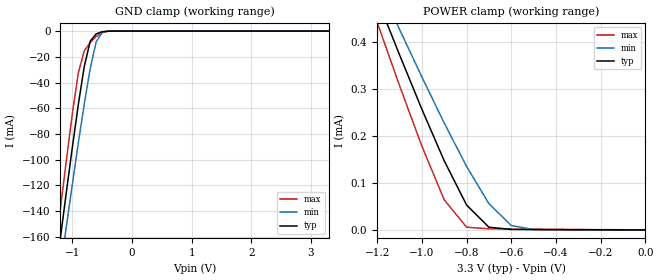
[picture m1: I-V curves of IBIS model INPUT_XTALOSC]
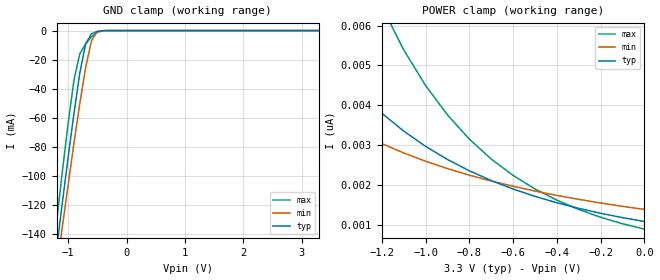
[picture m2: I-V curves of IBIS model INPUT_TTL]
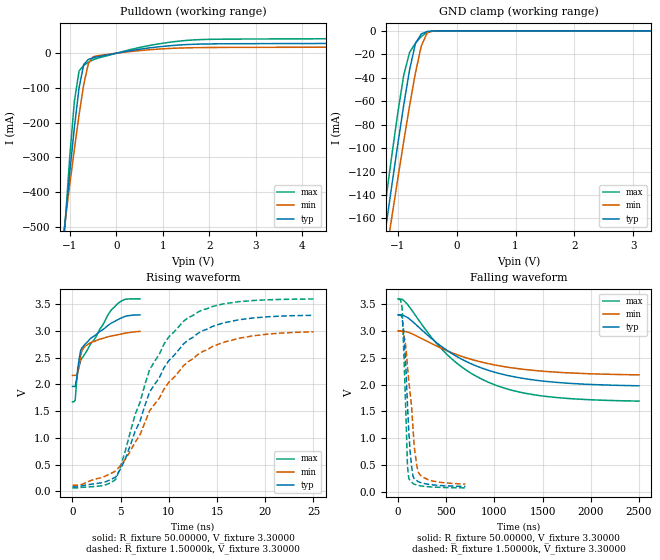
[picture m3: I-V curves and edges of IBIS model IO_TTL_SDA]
| IBIS file 5V19EE404.ibs created by s2ibis2 version 1.2
| North Carolina State University Electronics Research Laboratory  1995
[IBIS ver]   4.1
[File name]   5v19ee404.ibs
[File Rev]   2.7
[Date]   Aug 5, 2013
[Source]   IDT
[Notes]   1. Temp typ=25C, min=85C, max=-40C
[Disclaimer]
READ THESE TERMS AND CONDITIONS CAREFULLY BEFORE USING THIS IBIS MODEL.  BY
USING THIS IBIS MODEL, YOU ARE ACCEPTING AND AGREEING TO THESE TERMS AND
CONDITIONS OF USE.
Integrated Device Technology, Inc. ("IDT") hereby grants the user of this
IBIS model ("User") a non-exclusive, nontransferable license to use this
IBIS model under the following terms: The User is granted this license only
to use the IBIS model for demonstration purposes only and is not granted
rights to sell, copy (except as needed to run the IBIS model), rent, lease
or sub-license (except for demonstration) the IBIS model in whole or in
part, or in modified form to anyone. The User may modify the IBIS model to
suit its specific applications, but  rights to derivative works and such
modifications shall belong to IDT.
THIS IBIS MODEL IS PROVIDED ON AN AS IS" BASIS AND IDT  MAKES ABSOLUTELY NO
WARRANTY WITH RESPECT TO THE INFORMATION CONTAINED HEREIN.  IDT DISCLAIMS
AND USER WAIVES ALL WARRANTIES, EXPRESS AND IMPLIED, INCLUDING WARRANTIES OF
MERCHANTABILITY AND FITNESS FOR A PARTICULAR PURPOSE.  THE ENTIRE RISK AS TO
QUALITY AND PERFORMANCE IS WITH THE USER  ACCORDINGLY, IN NO EVENT SHALL IDT
BE LIABLE FOR ANY DIRECT OR INDIRECT DAMAGES, WHETHER IN CONTRACT OR TORT,
INCLUDING ANY LOST PROFITS OR OTHER INCIDENTAL, CONSEQUENTIAL, EXEMPLARY, OR
PUNITIVE DAMAGES ARISING OUT OF THE USE OR APPLICATION OF THE  IBIS MODEL,
WHETHER OR NOT IDT HAD NOTICE OF SUCH DAMAGES.
IDT reserves the right to make changes without notice to any product herein
to improve reliability, function, or design. IDT does not convey any license
under patent rights or any other intellectual property rights, including
those of third parties. IDT is not obligated to provide  maintenance or
support for the licensed IBIS model.
This model is for  IDT5V19EE404 IDT Programmable Clock
[Copyright]
Copyright 2002, Integrated Device Technology, Inc. All rights  reserved.
|History
|Rev 2.7 Updated on August 05, 2013   update RRef for TTL_SDA model
|Rev 2.6 Updated on Nov 01, 2012   update out4/4b 5/5b and single end output
|Rev 2.5 Updated on August 07, 2012   update diff table
|Rev 2.4 Updated on August 06, 2012   correct HCSL data error
|Rev 2.3 Updated on August 05, 2012   fix lvmos_1v8_s10 data error
|Rev 2.2 Updated on August 03, 2012   add lvcmos 1v8 output data
|Rev 2.1 Updated on August 02, 2012
|Rev 2.0 Updated on July 27, 2012
|Rev 1.0 Created on May 21, 2009
|   Component IDT5V19EE404
[Component]   IDT5V19EE404
[Manufacturer]   Integrated Device Technology Inc.
[Package]
| Following package parameters are for the 32 pin QFN package
| variable   typ   min   max
R_pkg   72.4655m   58.886m   86.045m
L_pkg   1.47175nH   1.11650nH   1.77850nH
C_pkg   0.07747pF   0.07444pF   0.08050pF
[Pin]  signal_name   model_name
1 vIN   POWER
2 XOUT   NC
3 XIN/REF   INPUT_XTALOSC
4 VDDx   POWER
5 CLKIN   INPUT_TTL
6 GND   GND
7 OUT1   lvcmos_se3
8 OUT2.   lvcmos_se3
9 VDDO1   POWER
10 VDD   POWER
11 SDAT   IO_TTL_SDA
12 SCLK   INPUT_TTL
13 CLKSEL   INPUT_TTL
14 AVDD   POWER
15 GND   GND
16 OUT6   lvcmos_se45
17 OUT3   lvcmos_se45
18 VDDO3   POWER
19 SEL2   INPUT_TTL
20 SEL1   INPUT_TTL
21 SEL0   INPUT_TTL
22 SD/OE   INPUT_TTL
23 GND   GND
24 VDD   POWER
[Diff Pin]  inv_pin  vdiff   tdelay_typ  tdelay_min  tdelay_max
11   10   0.000V   0.000s   0.000s   0.000s
15   14   0.000V   0.000s   0.000s   0.000s
[Model Selector] output_diff
output_lvds 3.3V LVDS output
output_lvpecl 3.3V LVPECL output
output_hcsl HCSL output
[Model Selector] lvcmos_se3
se3_1v8_s00 slew rate 00
se3_1v8_s01 slew rate 01
se3_1v8_s10 slew rate 10
se3_1v8_s11 slew rate 11
se3_3v3_s00 slew rate 00
se3_3v3_s01 slew rate 01
se3_3v3_s10 slew rate 10
se3_3v3_s11 slew rate 11
[Model Selector] lvcmos_se45
se45_1v8_s00 1.8v slew rate 00
se45_1v8_s01 1.8v slew rate 01
se45_1v8_s10 1.8v slew rate 10
se45_1v8_s11 1.8v slew rate 11
se45_3v3_s00 3.3v slew rate 00
se45_3v3_s01 3.3v slew rate 01
se45_3v3_s10 3.3v slew rate 10
se45_3v3_s11 3.3v slew rate 11
| Models and submodels in the file (22): INPUT_XTALOSC (Input), INPUT_TTL (Input), IO_TTL_SDA (I/O_open_drain), output_lvds (Output), output_lvpecl (Output_ECL), output_hcsl (Open_source), se45_1v8_s00 (Output), se45_1v8_s01 (Output), se45_1v8_s10 (Output), se45_1v8_s11 (Output), se45_3v3_s00 (Output), se45_3v3_s01 (Output), se45_3v3_s10 (Output), se45_3v3_s11 (Output), se3_1v8_s00 (Output), se3_1v8_s01 (Output), se3_1v8_s10 (Output), se3_1v8_s11 (Output), se3_3v3_s00 (Output), se3_3v3_s01 (Output), se3_3v3_s10 (Output), se3_3v3_s11 (Output)
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|   Model INPUT_XTALOSC
[Model]   INPUT_XTALOSC
Model_type   Input
Polarity   Non-Inverting
Vinl =  0.80000V
Vinh =  2.00000V
C_comp   4.00000pF   4.00000pF   4.00000pF
[Temperature Range]   25.00000   100.00000   -40.00000
[Voltage Range]   3.30000V   3.00000V   3.60000V
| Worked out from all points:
|   GND clamp passes 1 mA (typ) near -0.53 V on its own axis
|   POWER clamp passes 1 mA (typ) near -1.62 V on its own axis
[GND_clamp]
| voltage   I(typ)   I(min)   I(max)
-3.3V     -943.7mA   -911.4mA   -977.9mA
-1.3V     -196.5mA   -218.3mA   -176.1mA
-1.2V     -160.4mA   -184.7mA   -137.6mA
-1.1V     -124.9mA   -151.5mA   -99.98mA
-1V       -90.17mA   -118.9mA   -63.99mA
-900mV    -56.99mA   -87.01mA   -32.53mA
-800mV    -27.37mA   -56.54mA   -15.26mA
-700mV    -7.824mA   -28.91mA   -8.942mA
-600mV    -2.175mA   -8.303mA   -4.213mA
-500mV    -492.4uA   -874.3uA   -1.14mA
-400mV    -59.94uA   -63.48uA   -132.1uA
3.3V      67.86nA    72.43nA    13.64nA
[POWER_clamp]
| voltage   I(typ)   I(min)   I(max)
-3.3V     3.118mA    2.794mA    3.419mA
-1.2V     490.8uA    528.9uA    440.7uA
-1.1V     371.9uA    425.9uA    306.6uA
-1V       256.3uA    324.8uA    178uA
-900mV    146.8uA    227uA      63.96uA
-800mV    52.93uA    134.9uA    5.913uA
-700mV    5.782uA    55.77uA    2.388uA
-600mV    1.226uA    9.437uA    1.951uA
-500mV    889.4nA    759.8nA    1.591uA
0V        67.86nA    4.057nA    297.8nA
|   Model INPUT_TTL
[Model]   INPUT_TTL
Model_type   Input
Polarity   Non-Inverting
Vinl =  0.80000V
Vinh =  2.00000V
C_comp   3.15000pF   3.15000pF   3.15000pF
[Temperature Range]   25.00000   100.00000   -40.00000
[Voltage Range]   3.30000V   3.00000V   3.60000V
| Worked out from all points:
|   GND clamp passes 1 mA (typ) near -0.53 V on its own axis
[GND_clamp]
| voltage   I(typ)   I(min)   I(max)
-3.3V     -860.5mA   -813.9mA   -910.1mA
-1.3V     -183.6mA   -194.8mA   -167.8mA
-1.2V     -150.9mA   -164.8mA   -132.1mA
-1.1V     -118.6mA   -135.1mA   -97.13mA
-1V       -86.99mA   -105.9mA   -63.61mA
-900mV    -56.64mA   -77.31mA   -33.82mA
-800mV    -29.01mA   -50mA      -15.89mA
-700mV    -9.031mA   -25.22mA   -9.146mA
-600mV    -2.261mA   -6.881mA   -4.277mA
-500mV    -493.9uA   -650.7uA   -1.144mA
-400mV    -59.34uA   -43.85uA   -131.5uA
3.3V      1.08nA     1.636nA    591.5pA
[POWER_clamp]
| voltage   I(typ)   I(min)   I(max)
-3.3V     74.3nA     29.42nA    315.2nA
-1.9V     9.867nA    5.868nA    24.24nA
-1.6V     6.467nA    4.338nA    13.72nA
-1.5V     5.639nA    3.947nA    11.36nA
-1.4V     4.929nA    3.604nA    9.41nA
-1.2V     3.799nA    3.036nA    6.48nA
-1.1V     3.351nA    2.801nA    5.39nA
-1V       2.967nA    2.593nA    4.494nA
-900mV    2.637nA    2.408nA    3.756nA
-700mV    2.107nA    2.096nA    2.649nA
-400mV    1.55nA     1.735nA    1.615nA
0V        1.08nA     1.382nA    886.8pA
|   Model IO_TTL_SDA
[Model]   IO_TTL_SDA
Model_type   I/O_open_drain
Polarity   Non-Inverting
Vinl =  0.80000V
Vinh =  2.00000V
Vmeas =  1.65000V
Cref =   5.00pF
Rref =  500
Vref =   1.65V
C_comp   3.90000pF   3.90000pF   3.90000pF
[Temperature Range]   25.00000   100.00000   -40.00000
[Voltage Range]   3.30000V   3.00000V   3.60000V
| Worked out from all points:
|   slope of the pulldown table from 0 to 0.495 V, typ, clamps not added: 43.5 ohm
|   GND clamp passes 1 mA (typ) near -0.52 V on its own axis
|   rising waveform, R_fixture 50.00000, V_fixture 3.30000: 20-80 % time 2.7ns typ, 1.89ns min, 3.01ns max; typ from 1.96 V to 3.3 V
|   rising waveform, R_fixture 1.50000k, V_fixture 3.30000: 20-80 % time 5.32ns typ, 6.11ns min, 4.5ns max; typ from 0.084 V to 3.29 V
|   falling waveform, R_fixture 50.00000, V_fixture 3.30000: 20-80 % time 745ns typ, 797ns min, 692ns max; typ from 3.3 V to 1.98 V
|   falling waveform, R_fixture 1.50000k, V_fixture 3.30000: 20-80 % time 55.4ns typ, 83.7ns min, 39.4ns max; typ from 3.3 V to 0.098 V
[Pulldown]
| voltage   I(typ)   I(min)   I(max)
-3.3V     -3.766A    -2.968A    -5.052A
-1.3V     -769.4mA   -703.4mA   -881.9mA
-1V       -344.3mA   -379.3mA   -298.9mA
-900mV    -213.2mA   -275.9mA   -138.2mA
-800mV    -100.1mA   -177.7mA   -51.19mA
-700mV    -32.56mA   -90.56mA   -35.2mA
-600mV    -17.75mA   -30.02mA   -25.79mA
-500mV    -13.24mA   -10.47mA   -18.79mA
600mV     13.4mA     8.771mA    19.31mA
1.5V      24.87mA    15.54mA    36.84mA
5.1V      29.24mA    17.99mA    43.76mA
6.6V      42.47mA    25.45mA    67.13mA
[GND_clamp]
| voltage   I(typ)   I(min)   I(max)
-3.3V     -941mA     -907.6mA   -976.3mA
-1.3V     -202.4mA   -224.6mA   -181.6mA
-1.2V     -166.7mA   -191.4mA   -143.4mA
-1.1V     -131.5mA   -158.6mA   -106mA
-1V       -96.95mA   -126.3mA   -70.13mA
-900mV    -63.73mA   -94.63mA   -38.18mA
-800mV    -33.34mA   -64.12mA   -18.46mA
-700mV    -10.74mA   -35.84mA   -10.48mA
-600mV    -2.575mA   -12.79mA   -4.779mA
-500mV    -539.2uA   -1.691mA   -1.235mA
-400mV    -63.38uA   -109.7uA   -138.9uA
3.3V      1.086nA    4.119nA    592.1pA
[Ramp]
| variable   typ   min   max
dV/dt_r   1.92508/5.19520n   1.72182/6.10290n   2.11914/4.49638n
dV/dt_f   1.92147/55.29974n   1.71552/81.65226n   2.11722/40.58984n
R_load = 1.50000k
[Rising Waveform]
R_fixture = 50.00000
V_fixture = 3.30000
V_fixture_min = 3.00000
V_fixture_max = 3.60000
| Time   typ   min   max
0s        1.96V      2.167V     1.674V
280ps     1.961V     2.167V     1.703V
420ps     2.099V     2.171V     2.041V
560ps     2.318V     2.227V     2.253V
840ps     2.628V     2.535V     2.442V
980ps     2.685V     2.632V     2.491V
1.82ns    2.849V     2.774V     2.737V
3.78ns    3.115V     2.894V     3.327V
5.32ns    3.262V     2.952V     3.581V
7ns       3.299V     2.991V     3.599V
[Rising Waveform]
R_fixture = 1.50000k
V_fixture = 3.30000
V_fixture_min = 3.00000
V_fixture_max = 3.60000
| Time   typ   min   max
0s        83.54mV    113.3mV    64.1mV
4.5ns     268.8mV    380.5mV    223.7mV
5.5ns     615.4mV    601.9mV    769mV
6.5ns     1.121V     917.6mV    1.436V
7ns       1.309V     1.054V     1.66V
8ns       1.855V     1.503V     2.273V
10ns      2.446V     2.04V      2.89V
11.5ns    2.752V     2.344V     3.177V
16ns      3.163V     2.804V     3.515V
25ns      3.292V     2.982V     3.596V
[Falling Waveform]
R_fixture = 50.00000
V_fixture = 3.30000
V_fixture_min = 3.00000
V_fixture_max = 3.60000
| Time   typ   min   max
0s        3.3V       3V         3.6V
50ns      3.296V     2.998V     3.587V
100ns     3.251V     2.982V     3.494V
350ns     2.855V     2.763V     2.874V
550ns     2.588V     2.6V       2.49V
750ns     2.394V     2.475V     2.219V
950ns     2.259V     2.385V     2.034V
1.2us     2.147V     2.308V     1.885V
1.5us     2.066V     2.25V      1.786V
2.5us     1.976V     2.181V     1.69V
[Falling Waveform]
R_fixture = 1.50000k
V_fixture = 3.30000
V_fixture_min = 3.00000
V_fixture_max = 3.60000
| Time   typ   min   max
0s        3.3V       3V         3.6V
42ns      3.262V     2.996V     3.442V
70ns      2.688V     2.847V     2.087V
98ns      1.611V     2.341V     473.4mV
112ns     1.111V     2.056V     243.5mV
140ns     485.4mV    1.603V     179.4mV
154ns     296mV      1.221V     155.3mV
168ns     242.8mV    847.9mV    138.9mV
210ns     186.7mV    363.7mV    115.8mV
700ns     97.55mV    140.8mV    71.3mV
